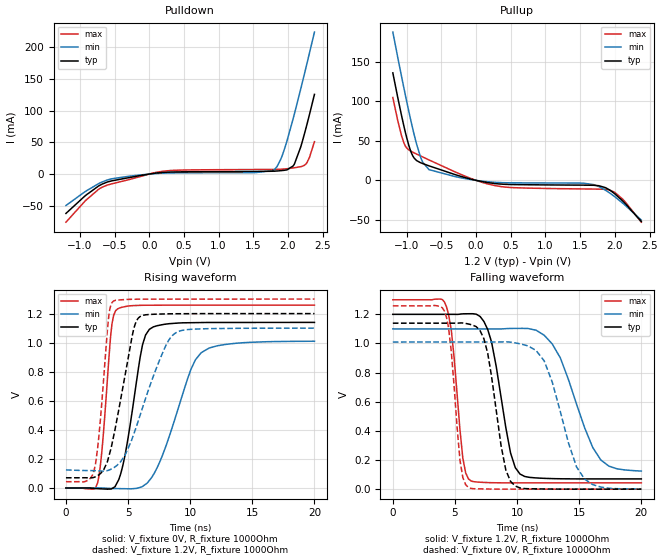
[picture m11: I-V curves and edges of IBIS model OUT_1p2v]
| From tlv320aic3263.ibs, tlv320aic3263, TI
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|   OUT_1p2v
[Model]   OUT_1p2v
Model_type   Output
Polarity   Non-Inverting
Vmeas = 0.6
Vref = 0
Cref = 5pF
Rref = 10000
|   typ   min   max
C_comp   1.397pF   1.384pF   1.430pF
[Voltage Range]   1.2   1.1   1.3
[Temperature Range]   27   125   -40
[Pullup Reference]   1.2   1.1   1.3
[Pulldown Reference]   -0   -0   -0
[Power Clamp Reference]   1.2   1.1   1.3
[GND Clamp Reference]   -0   -0   -0
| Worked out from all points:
|   slope of the pulldown table from 0 to 0.18 V, typ, clamps not added: 75.7 ohm
|   slope of the pullup table from 0 to 0.18 V, typ, clamps not added: 60.4 ohm
|   falling waveform, V_fixture 1.2V, R_fixture 1000Ohm: 20-80 % time 1.34ns typ, 2.47ns min, 778ps max; typ from 1.2 V to 0.07 V
|   rising waveform, V_fixture 0V, R_fixture 1000Ohm: 20-80 % time 1.24ns typ, 2.36ns min, 671ps max; typ from 0 V to 1.14 V
|   rising waveform, V_fixture 1.2V, R_fixture 1000Ohm: 20-80 % time 1.49ns typ, 2.41ns min, 725ps max; typ from 0.07 V to 1.2 V
|   falling waveform, V_fixture 0V, R_fixture 1000Ohm: 20-80 % time 1.19ns typ, 2.08ns min, 728ps max; typ from 1.14 V to 0 V
[Pulldown]
|   Voltage   I(typ)   I(min)   I(max)
-1.2V     -62.16mA   -49.66mA   -76.01mA
-912mV    -33.33mA   -26.93mA   -41.32mA
-696mV    -16.83mA   -13.35mA   -21.8mA
42mV      706.8uA    400uA      1.221mA
420mV     3.439mA    1.921mA    6.168mA
1.788V    4.491mA    5.813mA    7.278mA
1.842V    4.86mA     11.68mA    7.389mA
1.914V    5.538mA    28.27mA    7.763mA
2.094V    16.09mA    95.4mA     9.969mA
2.184V    42.72mA    134.3mA    11.7mA
2.274V    78.52mA    174.6mA    18.06mA
2.382V    125.8mA    224.2mA    51.12mA
[Pullup]
|   Voltage   I(typ)   I(min)   I(max)
-1.2V     135.9mA    187.5mA    104.8mA
-1.128V   104.4mA    155.1mA    75.15mA
-1.038V   67.66mA    115.8mA    46.82mA
-930mV    34.2mA     71.68mA    36.39mA
-804mV    22.46mA    30.45mA    31.04mA
-678mV    18.35mA    13.53mA    25.8mA
-84mV     1.789mA    1.133mA    2.732mA
312mV     -4.378mA   -2.645mA   -7.186mA
1.554V    -6.04mA    -3.598mA   -10.86mA
1.77V     -6.748mA   -7.833mA   -11.06mA
2.004V    -17.36mA   -21mA      -15.52mA
2.382V    -52.03mA   -50.29mA   -52.89mA
[Ramp]
R_load = 1000
|   typ   min   max
dV/dt_r   0.683622/1.2416e-009   0.605093/2.36124e-009   0.75487/6.71419e-010
dV/dt_f   0.677798/1.3438e-009   0.585475/2.47368e-009  0.754006/7.78483e-010
[Falling Waveform]
V_fixture = 1.2V
V_fixture_min = 1.1V
V_fixture_max = 1.3V
R_fixture = 1000Ohm
C_fixture = 0F
|   Time   V(typ)   V(min)   V(max)
0s        1.2V       1.1V       1.3V
4.315ns   1.2V       1.1V       1.252V
4.707ns   1.2V       1.1V       1.092V
5.632ns   1.203V     1.1V       213.3mV
6.095ns   1.204V     1.1V       69.28mV
7.639ns   1.095V     1.1V       45.18mV
10.24ns   103.4mV    1.104V     43.27mV
12.83ns   72.51mV    996.5mV    43.32mV
16.74ns   70.34mV    200.1mV    43.32mV
20ns      70.34mV    124.2mV    43.32mV
[Rising Waveform]
V_fixture = 0V
V_fixture_min = 0V
V_fixture_max = 0V
R_fixture = 1000Ohm
C_fixture = 0F
|   Time   V(typ)   V(min)   V(max)
0s        -828.9nV   1.32mV     185.5pV
2.541ns   -4.667mV   719.1uV    33.57mV
2.942ns   -6.35mV    -100.2uV   302mV
3.706ns   -3.787mV   -3.485mV   1.13V
4.155ns   42.37mV    -4.11mV    1.232V
4.83ns    260.9mV    -5.048mV   1.249V
6.161ns   985.1mV    10.72mV    1.257V
6.715ns   1.092V     52.47mV    1.258V
10.88ns   1.138V     930.6mV    1.258V
20ns      1.139V     1.01V      1.258V
[Rising Waveform]
V_fixture = 1.2V
V_fixture_min = 1.1V
V_fixture_max = 1.3V
R_fixture = 1000Ohm
C_fixture = 0F
|   Time   V(typ)   V(min)   V(max)
0s        70.34mV    124.2mV    43.32mV
2.251ns   73.29mV    119.4mV    114.6mV
2.7ns     94.2mV     117.4mV    402.2mV
3.452ns   217.4mV    123.1mV    1.187V
3.835ns   355.8mV    138.9mV    1.287V
5.427ns   1.084V     363.8mV    1.299V
5.968ns   1.18V      500.8mV    1.299V
7.792ns   1.197V     932.8mV    1.3V
8.91ns    1.199V     1.071V     1.3V
20ns      1.2V       1.1V       1.3V
[Falling Waveform]
|Gnd
V_fixture = 0V
V_fixture_min = 0V
V_fixture_max = 0V
R_fixture = 1000Ohm
C_fixture = 0F
|   Time   V(typ)   V(min)   V(max)
0s        1.139V     1.01V      1.258V
4.155ns   1.139V     1.01V      1.222V
5.401ns   1.141V     1.01V      200.6mV
6.095ns   1.133V     1.01V      10.98mV
7.331ns   1.033V     1.01V      1.456mV
9.093ns   131.6mV    1.011V     43.01uV
9.857ns   21.36mV    1.004V     -26.22uV
12.18ns   1.322mV    880.7mV    -20.21uV
15.44ns   36.92uV    68.66mV    -11.79uV
20ns      -726.5nV   1.306mV    -599.7pV
